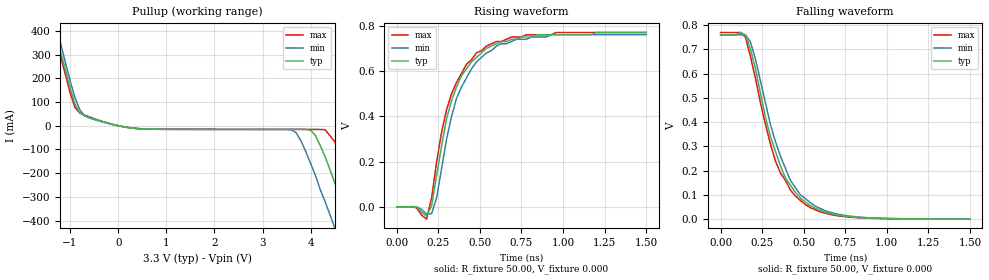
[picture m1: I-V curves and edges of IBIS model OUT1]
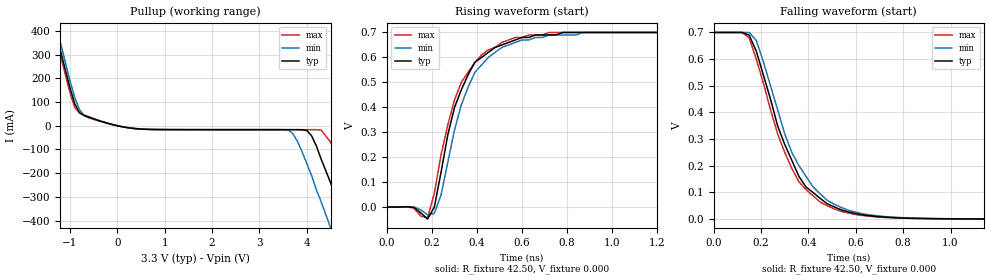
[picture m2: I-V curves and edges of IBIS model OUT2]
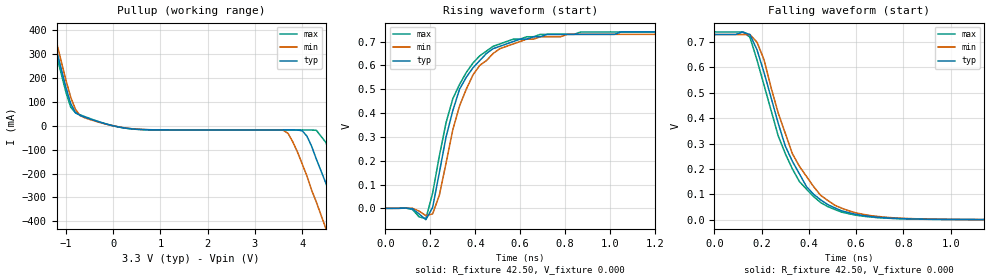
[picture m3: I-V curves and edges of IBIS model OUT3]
| Integrated Devices Technolgy, Inc
[Ibis Ver]   3.2
[File Name]   9zx21501b.ibs
[File Rev]   1.1
[Date]   5/20/2009
|[Date]   [File Rev] 1.0 Tuesday, September 30, 2008
[Source]   Integrated Devices Technolgy, Inc.
|[Notes]   Rev 1.0 created by yfeng
[Notes]   Rev 1.1 added Vref, Rref, Vmeas
[Disclaimer] Integrated Device Technology, Inc. ("IDT") hereby grants the
   user of this IBIS model a non-exclusive, nontransferable
   license to use this IBIS model under the following terms. The
   user is granted this license only to use the IBIS model and is
   not granted rights to sell, copy (except as needed to run the
   IBIS model), rent, lease or sub-license the IBIS model in
   whole or in part, or in modified form to anyone. The User may
   modify the IBIS model to suit its specific applications, but
   rights to derivative works and such modifications shall belong
   to IDT. This IBIS model is provided on an AS IS" basis and IDT
   makes absolutely no warranty with respect to the information
   contained herein. IDT DISCLAIMS AND CUSTOMER WAIVES ALL
   WARRANTIES, EXPRESS AND IMPLIED, INCLUDING WARRANTIES OF
   MERCHANTABILITY AND FITNESS FOR A PARTICULAR PURPOSE. THE
   ENTIRE RISK AS TO QUALITY AND PERFORMANCE IS WITH THE USER
   ACCORDINGLY, IN NO EVENT SHALL IDT BE LIABLE FOR ANY DIRECT OR
   INDIRECT DAMAGES, WHETHER IN CONTRACT OR TORT, INCLUDING ANY
   LOST PROFITS OR OTHER INCIDENTAL, CONSEQUENTIAL, EXEMPLARY, OR
   PUNITIVE DAMAGES ARISING OUT OF THE USE OR APPLICATION OF THE
   IBIS model. Further, IDT reserves the right to make changes
   without notice to any product herein to improve reliability,
   function, or design. IDT does not convey any license under
   patent rights or any other intellectual property rights,
   including those of third parties. IDT is not obligated to
   provide maintenance or support for the licensed IBIS model.
[Disclaimer]   (C) Copyright Integrated Device Technology, Inc. 2007 All
   rights reserved
|   COMPONENT: ICS9ZX21501
[Component]   ICS9ZX21501
[Manufacturer]   Integrated Device Technology, Inc.
[Package]
| variable   typ   min   max
R_pkg   81.10m   62.20m   100.00m
L_pkg   6.70nH   4.90nH   8.50nH
C_pkg   0.53pF   0.21pF   0.85pF
[Pin]   signal_name   model_name   R_pin   L_pin   C_pin
1   IREF   OUT
2   100M_133M#   IN
3   HIBW_BYPM_LOBW#   IN
4   CK_POWERGD/PD#   IN
5   GND   GND
6   VDD   POWER
7   DIF_IN   IN
8   DIF_IN#   IN
9   SMB_A0_tri   IN
10   SMBDAT   IO_D
11   SMBCLK   IN_D
12   SMB_A1_tri   IN
13   DFB_IN   IN
14   DFB_IN#   IN
15   DFB_OUT#   OUT
16   DFB_OUT   OUT
17   DIF_0   OUT
18   DIF_0#   OUT
19   VDD   POWER
20   DIF_1   OUT
21   DIF_1#   OUT
22   DIF_2   OUT
23   DIF_2#   OUT
24   GND   GND
25   DIF_4   OUT
26   DIF_4#   OUT
27   VDD   POWER
28   DIF_5   OUT
29   DIF_5#   OUT
30   OE5#   IN
31   DIF_6   OUT
32   DIF_6#   OUT
33   OE6#   IN
34   DIF_7   OUT
35   DIF_7#   OUT
36   OE7#   IN
37   DIF_8   OUT
38   DIF_8#   OUT
39   OE8#   IN
40   GND   GND
41   VDD   POWER
42   NC   NC
43   DIF_10   OUT
44   DIF_10#   OUT
45   OE10#   IN
46   DIF_11   OUT
47   DIF_11#   OUT
48   OE_11#   IN
49   DIF_12   OUT
50   DIF_12#   OUT
51   OE12#   IN
52   VDD   POWER
53   DIF_13   OUT
54   DIF_13#   OUT
55   GND   GND
56   DIF_15   OUT
57   DIF_15#   OUT
58   DIF_16   OUT
59   DIF_16#   OUT
60   VDD   POWER
61   DIF_17   OUT
62   DIF_17#   OUT
63   VDDA   POWER
64   GNDA   GND
[Diff Pin]   inv_pin   vdiff   tdelay_typ
16   15   NA   NA
17   18   NA   NA
20   21   NA   NA
22   23   NA   NA
25   26   NA   NA
28   29   NA   NA
31   32   NA   NA
34   35   NA   NA
37   38   NA   NA
43   44   NA   NA
46   47   NA   NA
49   50   NA   NA
53   54   NA   NA
56   57   NA   NA
58   59   NA   NA
61   62   NA   NA
[Model Selector] OUT
OUT1   100ohm differential output trace. 475ohm on IREF pin.
OUT2   85ohm differential output trace. 432ohm on IREF pin.
OUT3   85ohm differential output trace. 412ohm on IREF pin.
| Models and submodels in the file (6): OUT1 (Open_source), OUT2 (Open_source), OUT3 (Open_source), IN (Input), IO_D (I/O_open_drain), IN_D (Input)
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|   Model OUT1
[Model]   OUT1
Model_type   Open_source
Polarity   Non-Inverting
Vmeas =  0.350V
Cref =   2.00pF
Rref =  50.000
Vref =   0.350V
Enable   Active-High
C_comp   3.40pF   2.85pF   3.95pF
[Temperature Range]   27.00   70.00   0.000
[Voltage Range]   3.30V   3.00V   3.60V
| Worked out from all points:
|   slope of the pullup table from 0 to 0.495 V, typ, clamps not added: 37.6 ohm
|   rising waveform, R_fixture 50.00, V_fixture 0.000: 20-80 % time 183ps typ, 183ps min, 178ps max; typ from 0 V to 0.77 V
|   falling waveform, R_fixture 50.00, V_fixture 0.000: 20-80 % time 194ps typ, 201ps min, 196ps max; typ from 0.76 V to 0 V
[Pullup]
| voltage   I(typ)   I(min)   I(max)
-3.3V     2.06A      2.09A      2.05A
-1.5V     550mA      590mA      530mA
-900mV    93.18mA    120mA      77.76mA
-500mV    28.45mA    26.28mA    30.19mA
3.6V      -15.31mA   -16.83mA   -15.36mA
4V        -18.89mA   -160mA     -15.37mA
4.3V      -130mA     -320mA     -16.85mA
4.5V      -240mA     -430mA     -67.51mA
4.7V      -350mA     -540mA     -170mA
4.9V      -460mA     -650mA     -280mA
5.1V      -580mA     -760mA     -400mA
6.6V      -1.44A     -1.6A      -1.27A
[Ramp]
| variable   typ   min   max
dV/dt_r   0.46/0.18n   0.46/0.18n   0.46/0.17n
dV/dt_f   0.46/0.20n   0.46/0.20n   0.46/0.19n
R_load = 50.00
[Rising Waveform]
R_fixture = 50.00
V_fixture = 0.000
V_fixture_min = 0.000
V_fixture_max = 0.000
| time   V(typ)   V(min)   V(max)
0s        52.45uV    49.42uV    57.25uV
120ps     -1.48mV    500uV      -4.67mV
180ps     -39.8mV    -32.47mV   -53.51mV
210ps     5.66mV     -29.54mV   41.27mV
240ps     140mV      40.56mV    200mV
300ps     390mV      300mV      430mV
360ps     530mV      480mV      550mV
480ps     660mV      640mV      680mV
720ps     740mV      740mV      750mV
1.5ns     770mV      760mV      770mV
[Falling Waveform]
R_fixture = 50.00
V_fixture = 0.000
V_fixture_min = 0.000
V_fixture_max = 0.000
| time   V(typ)   V(min)   V(max)
0s        760mV      760mV      770mV
120ps     770mV      760mV      770mV
150ps     760mV      760mV      750mV
180ps     700mV      730mV      670mV
270ps     420mV      480mV      390mV
330ps     280mV      320mV      240mV
420ps     140mV      160mV      120mV
510ps     70.41mV    84.41mV    60.12mV
780ps     9.22mV     11.83mV    7.74mV
1.5ns     66.75uV    97.12uV    35.69uV
|   Model OUT2
[Model]   OUT2
Model_type   Open_source
Polarity   Non-Inverting
Enable   Active-High
Vmeas =  0.350V
Cref =   2.00pF
Rref =  50.000
Vref =   0.350V
C_comp   3.40pF   2.85pF   3.95pF
[Temperature Range]   27.00   70.00   0.000
[Voltage Range]   3.30V   3.00V   3.60V
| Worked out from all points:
|   slope of the pullup table from 0 to 0.495 V, typ, clamps not added: 35.5 ohm
|   rising waveform, R_fixture 42.50, V_fixture 0.000: 20-80 % time 138ps typ, 149ps min, 149ps max; typ from 0 V to 0.7 V
|   falling waveform, R_fixture 42.50, V_fixture 0.000: 20-80 % time 172ps typ, 185ps min, 167ps max; typ from 0.7 V to 0 V
[Pullup]
| voltage   I(typ)   I(min)   I(max)
-3.3V     2.06A      2.09A      2.05A
-1.5V     550mA      590mA      530mA
-900mV    93.48mA    120mA      78.18mA
-500mV    28.92mA    26.72mA    30.68mA
500mV     -13.95mA   -13.46mA   -14.27mA
3.6V      -16.51mA   -18.02mA   -16.56mA
4V        -20.09mA   -160mA     -16.57mA
4.3V      -140mA     -320mA     -18.05mA
4.5V      -240mA     -430mA     -68.71mA
4.9V      -470mA     -650mA     -280mA
5.1V      -580mA     -760mA     -400mA
6.6V      -1.44A     -1.6A      -1.27A
[Ramp]
| variable   typ   min   max
dV/dt_r   0.49/0.18n   0.49/0.19n   0.50/0.18n
dV/dt_f   0.49/0.19n   0.49/0.20n   0.50/0.19n
R_load = 50.00
[Rising Waveform]
R_fixture = 42.50
V_fixture = 0.000
V_fixture_min = 0.000
V_fixture_max = 0.000
| time   V(typ)   V(min)   V(max)
0s        51.6uV     48.65uV    56.35uV
120ps     -1.67mV    460uV      -5.05mV
180ps     -48.04mV   -31.16mV   -42.6mV
210ps     -550uV     -25.45mV   54.69mV
270ps     290mV      180mV      330mV
330ps     470mV      410mV      500mV
390ps     580mV      540mV      580mV
510ps     650mV      640mV      660mV
870ps     700mV      700mV      700mV
1.5ns     700mV      700mV      700mV
[Falling Waveform]
R_fixture = 42.50
V_fixture = 0.000
V_fixture_min = 0.000
V_fixture_max = 0.000
| time   V(typ)   V(min)   V(max)
0s        700mV      700mV      700mV
120ps     700mV      700mV      700mV
150ps     690mV      700mV      680mV
180ps     630mV      670mV      600mV
270ps     350mV      410mV      320mV
330ps     220mV      250mV      190mV
390ps     120mV      160mV      110mV
450ps     77.34mV    94.08mV    63.61mV
720ps     7.36mV     9.45mV     6.14mV
1.5ns     41.6uV     45.49uV    -5.31uV
|   Model OUT3
[Model]   OUT3
Model_type   Open_source
Polarity   Non-Inverting
Enable   Active-High
Vmeas =  0.350V
Cref =   2.00pF
Rref =  50.000
Vref =   0.350V
C_comp   3.40pF   2.85pF   3.95pF
[Temperature Range]   27.00   70.00   0.000
[Voltage Range]   3.30V   3.00V   3.60V
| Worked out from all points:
|   slope of the pullup table from 0 to 0.495 V, typ, clamps not added: 34.2 ohm
|   rising waveform, R_fixture 42.50, V_fixture 0.000: 20-80 % time 152ps typ, 148ps min, 150ps max; typ from 0 V to 0.74 V
|   falling waveform, R_fixture 42.50, V_fixture 0.000: 20-80 % time 172ps typ, 185ps min, 171ps max; typ from 0.73 V to 0 V
[Pullup]
| voltage   I(typ)   I(min)   I(max)
-3.3V     2.06A      2.09A      2.05A
-1.5V     550mA      590mA      530mA
-900mV    93.67mA    120mA      78.44mA
-500mV    29.22mA    26.99mA    31mA
500mV     -14.45mA   -13.92mA   -14.8mA
3.6V      -17.3mA    -18.82mA   -17.36mA
4V        -20.89mA   -160mA     -17.37mA
4.3V      -140mA     -320mA     -18.85mA
4.5V      -240mA     -430mA     -69.51mA
4.9V      -470mA     -650mA     -280mA
5.1V      -580mA     -760mA     -400mA
6.6V      -1.44A     -1.61A     -1.27A
[Ramp]
| variable   typ   min   max
dV/dt_r   0.52/0.19n   0.52/0.19n   0.52/0.18n
dV/dt_f   0.52/0.20n   0.52/0.20n   0.52/0.19n
R_load = 50.00
[Rising Waveform]
R_fixture = 42.50
V_fixture = 0.000
V_fixture_min = 0.000
V_fixture_max = 0.000
| time   V(typ)   V(min)   V(max)
0s        51.6uV     48.65uV    56.35uV
120ps     -1.67mV    460uV      -4.69mV
180ps     -47.48mV   -30.79mV   -43.47mV
210ps     3.73mV     -23.28mV   63.75mV
270ps     300mV      190mV      360mV
330ps     500mV      430mV      520mV
390ps     590mV      560mV      610mV
480ps     670mV      650mV      680mV
810ps     730mV      730mV      730mV
1.5ns     740mV      730mV      740mV
[Falling Waveform]
R_fixture = 42.50
V_fixture = 0.000
V_fixture_min = 0.000
V_fixture_max = 0.000
| time   V(typ)   V(min)   V(max)
0s        730mV      730mV      740mV
120ps     740mV      730mV      740mV
150ps     730mV      730mV      720mV
180ps     670mV      700mV      630mV
270ps     380mV      420mV      330mV
330ps     230mV      260mV      200mV
390ps     130mV      170mV      120mV
480ps     59.35mV    75.72mV    51.54mV
750ps     6mV        7.86mV     4.91mV
1.5ns     58.66uV    38.86uV    990nV
